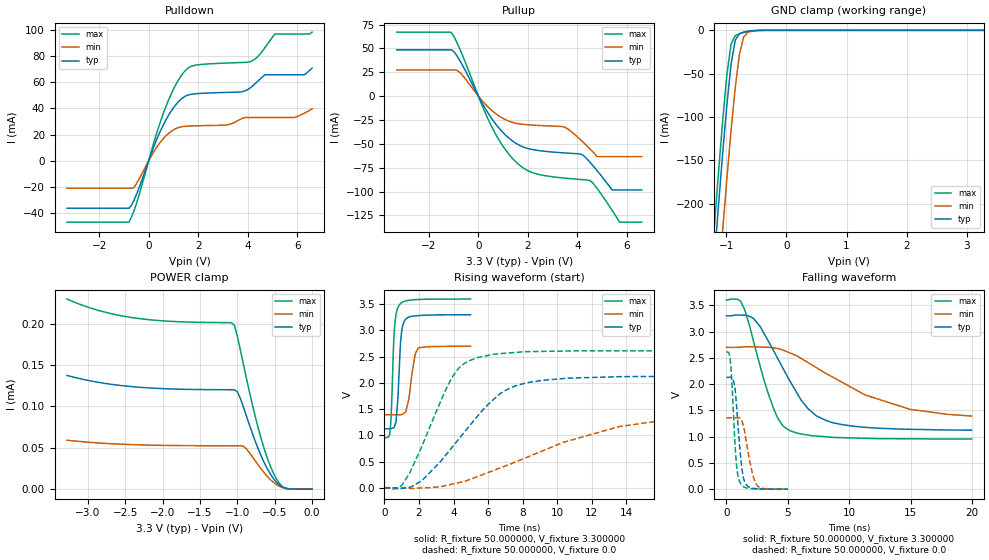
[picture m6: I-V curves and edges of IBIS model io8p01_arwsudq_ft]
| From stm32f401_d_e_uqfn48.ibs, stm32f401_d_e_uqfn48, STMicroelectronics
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|   Model io8p01_arwsudq_ft
[Model]  io8p01_arwsudq_ft
Model_type I/O
Polarity   Non-Inverting
Enable   Active-Low
Vinl =   0.990000V
Vinh =   2.310000V
Vmeas =  1.650000V
Cref =   50.000000pF
Rref =   100.000000M
Vref =   0.0V
C_comp   2.905500pF   2.823600pF   2.987900pF
[Temperature Range]   25.000000   0.125000k   -40.000000
[Pullup Reference]   3.300000V   2.700000V   3.600000V
[Pulldown Reference]   0.0V   0.0V   0.0V
[POWER Clamp Reference]   3.300000V   2.700000V   3.600000V
[GND Clamp Reference]   0.0V   0.0V   0.0V
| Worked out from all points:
|   slope of the pulldown table from 0 to 0.495 V, typ, clamps not added: 20.9 ohm
|   slope of the pullup table from 0 to 0.495 V, typ, clamps not added: 22.6 ohm
|   GND clamp passes 1 mA (typ) near -0.62 V on its own axis
|   rising waveform, R_fixture 50.000000, V_fixture 3.300000: 20-80 % time 213ps typ, 338ps min, 189ps max; typ from 1.12 V to 3.3 V
|   rising waveform, R_fixture 50.000000, V_fixture 0.0: 20-80 % time 3.35ns typ, 6.88ns min, 2.1ns max; typ from 0 V to 2.13 V
|   falling waveform, R_fixture 50.000000, V_fixture 3.300000: 20-80 % time 3.25ns typ, 6.72ns min, 2.01ns max; typ from 3.3 V to 1.12 V
|   falling waveform, R_fixture 50.000000, V_fixture 0.0: 20-80 % time 461ps typ, 655ps min, 374ps max; typ from 2.13 V to 0 V
[Pulldown]
|Voltage   I(typ)   I(min)   I(max)
-3.3V     -36.4mA    -21.08mA   -47.09mA
-800mV    -36.4mA    -21.08mA   -47.09mA
-600mV    -30.5mA    -20.54mA   -38.69mA
700mV     31.4mA     19.11mA    41.71mA
1.2V      45.15mA    25.37mA    61.75mA
1.6V      50.35mA    26.5mA     71.06mA
3.1V      52.28mA    27.26mA    74.76mA
4.1V      55.71mA    33.04mA    75.8mA
4.7V      65.81mA    33.04mA    86.69mA
5.1V      65.81mA    33.04mA    97.04mA
6.3V      65.87mA    36.5mA     97.04mA
6.6V      70.93mA    39.72mA    98.49mA
[Pullup]
|Voltage   I(typ)   I(min)   I(max)
-3.3V     48.56mA    27.45mA    67.2mA
-1.1V     48.56mA    27.45mA    66.91mA
-700mV    35.13mA    23.48mA    46.33mA
500mV     -22.07mA   -14mA      -30.03mA
1.5V      -49.1mA    -28.3mA    -68.56mA
2.2V      -56.05mA   -30.32mA   -80.35mA
3.5V      -59.53mA   -32.66mA   -85.92mA
4.5V      -69.08mA   -55.13mA   -88.39mA
4.8V      -78.24mA   -63.4mA    -96.88mA
5.4V      -98.3mA    -63.4mA    -119.6mA
5.7V      -98.3mA    -63.4mA    -132.1mA
6.6V      -98.3mA    -63.4mA    -132.1mA
[GND_clamp]
|Voltage   I(typ)   I(min)   I(max)
-3.3V     -2.319A    -2.397A    -2.292A
-1.2V     -266mA     -356.2mA   -228.4mA
-1.13V    -203.2mA   -293mA     -165.3mA
-1.06V    -142.7mA   -231.3mA   -105.2mA
-990mV    -86.51mA   -171.7mA   -51.78mA
-920mV    -39.3mA    -115.7mA   -15.93mA
-850mV    -11.37mA   -65.76mA   -6.097mA
-780mV    -3.83mA    -27.55mA   -3.88mA
-710mV    -2.09mA    -7.747mA   -2.382mA
-640mV    -1.147mA   -2.129mA   -1.22mA
-570mV    -523.9uA   -800uA     -476.9uA
3.28V     0A         0A         0A
[POWER_clamp]
|Voltage   I(typ)   I(min)   I(max)
-3.28V    137.3uA    59.14uA    229.6uA
-2.36V    123.4uA    53.65uA    206.6uA
-1.08V    120.1uA    52.41uA    201.1uA
-1.04V    120uA      52.41uA    198uA
-1V       117.7uA    52.4uA     184.5uA
-920mV    99.46uA    51.91uA    151.2uA
-720mV    48.42uA    29.12uA    73.51uA
-600mV    24.82uA    15.47uA    37.72uA
-520mV    13.1uA     8.45uA     19.84uA
-440mV    5.058uA    3.61uA     7.276uA
-360mV    1.193uA    1.129uA    1.311uA
0V        0A         0A         0A
[Ramp]
| variable   typ   min   max
dV/dt_r  1.27752/3.34417n   0.79896/6.88378n   1.56815/2.10146n
dV/dt_f  1.30248/3.25751n   0.74040/6.66937n   1.58786/2.00785n
R_load = 50.000000
[Rising Waveform]
R_fixture= 50.000000
V_fixture= 3.300000
V_fixture_min= 2.700000
V_fixture_max= 3.600000
|time   V(typ)   V(min)   V(max)
0s        1.124V     1.392V     954.3mV
300.3ps   1.126V     1.392V     1.012V
370.4ps   1.127V     1.392V     1.254V
570.6ps   1.159V     1.392V     2.999V
670.7ps   1.271V     1.391V     3.306V
830.8ps   2.084V     1.392V     3.47V
981ps     2.945V     1.394V     3.527V
1.241ns   3.22V      1.455V     3.563V
1.962ns   3.283V     2.668V     3.591V
4.985ns   3.3V       2.7V       3.599V
[Rising Waveform]
R_fixture= 50.000000
V_fixture= 0.0
V_fixture_min= 0.0
V_fixture_max= 0.0
|time   V(typ)   V(min)   V(max)
0s        360.6uV    205.5uV    689.3uV
1.001ns   -14.87mV   -990uV     47.26mV
2.162ns   132.8mV    -2.676mV   787mV
3.964ns   790.2mV    71.54mV    2.127V
4.565ns   1.034V     116.6mV    2.355V
5.325ns   1.341V     204.9mV    2.476V
6.767ns   1.809V     385.4mV    2.559V
8.408ns   2.011V     601.6mV    2.596V
13.61ns   2.118V     1.167V     2.611V
19.94ns   2.129V     1.359V     2.612V
[Falling Waveform]
R_fixture= 50.000000
V_fixture= 3.300000
V_fixture_min= 2.700000
V_fixture_max= 3.600000
|time   V(typ)   V(min)   V(max)
0s        3.3V       2.7V       3.599V
920.9ps   3.315V     2.7V       3.611V
1.481ns   3.31V      2.711V     3.419V
2.202ns   3.251V     2.71V      2.817V
3.764ns   2.666V     2.69V      1.582V
5.005ns   2.124V     2.608V     1.134V
6.687ns   1.521V     2.402V     1.027V
8.569ns   1.271V     2.143V     988.5mV
14.93ns   1.14V      1.52V      958.5mV
19.94ns   1.124V     1.392V     954.3mV
[Falling Waveform]
R_fixture= 50.000000
V_fixture= 0.0
V_fixture_min= 0.0
V_fixture_max= 0.0
|time   V(typ)   V(min)   V(max)
0s        2.129V     1.359V     2.612V
300.3ps   2.13V      1.359V     2.482V
620.6ps   2.024V     1.358V     1.2V
820.8ps   1.596V     1.36V      457.3mV
1.091ns   768.2mV    1.352V     134.1mV
1.291ns   334.4mV    1.28V      63.84mV
1.481ns   140.9mV    1.093V     36.31mV
2.142ns   17.53mV    269.8mV    7.487mV
2.452ns   9.451mV    85.43mV    5.303mV
4.985ns   360.6uV    205.5uV    689.3uV
